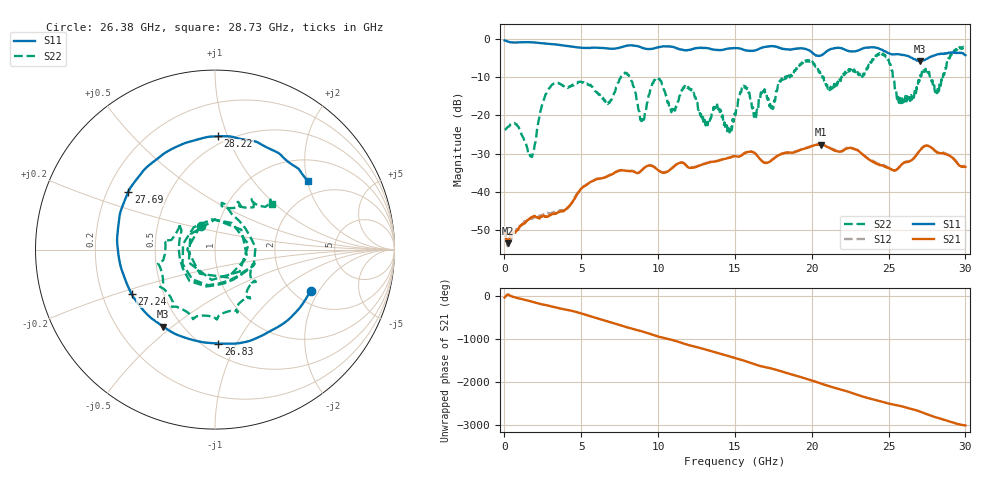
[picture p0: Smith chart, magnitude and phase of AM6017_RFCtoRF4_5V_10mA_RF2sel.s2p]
!Agilent Technologies,E8364B,MY43040894,A.07.50.67
!Agilent E8364B: A.07.50.67
!Date: Tuesday, August 21, 2018 13:31:20
!Correction: S11(Full 2 Port(1,2))
!S21(Full 2 Port(1,2))
!S12(Full 2 Port(1,2))
!S22(Full 2 Port(1,2))
!S2P File: Measurements: S11, S21, S12, S22:
# Hz S  dB  R 50
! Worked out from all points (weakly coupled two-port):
!   1601 points, 10 MHz to 30 GHz, reference 50 ohm
!   highest |S21| = -27.63 dB at 20.57 GHz (marker M1); lowest = -53.5 dB at 253.7 MHz (marker M2)
!   lowest |S11| = -5.7 dB at 27.06 GHz (marker M3), VSWR 3.14, Z = 19.9 - j23.2 ohm
!   |S11| at or under -10 dB: nowhere
!   |S22| runs from -30.9 to -1.7 dB; largest |S21 - S12| = 0.0061
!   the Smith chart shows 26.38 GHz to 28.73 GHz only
!   S11 on the Smith chart (normalised r, x): 26.38 GHz: 2.45, -1.69; 26.83 GHz: 0.59, -0.85; 27.24 GHz: 0.33, -0.22; 27.69 GHz: 0.29, +0.28; 28.22 GHz: 0.44, +0.92; 28.73 GHz: 1.55, +2.02
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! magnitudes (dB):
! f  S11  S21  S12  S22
! 10 MHz  -0.4  -50.1  -50.4  -23.7
! 253.7 MHz  -0.7  -53.5  -53.9  -23.0
! 1.772 GHz  -0.9  -46.7  -47.1  -30.9
! 2.934 GHz  -1.3  -46.2  -45.7  -12.8
! 5.015 GHz  -2.3  -39.1  -39.1  -11.2
! 6.739 GHz  -2.5  -35.9  -35.8  -17.0
! 7.957 GHz  -1.7  -34.6  -34.5  -8.9
! 8.97 GHz  -2.3  -34.2  -34.2  -21.9
! 10.02 GHz  -2.2  -34.4  -34.4  -10.4
! 10.96 GHz  -2.1  -33.6  -33.6  -19.0
! 15.01 GHz  -2.4  -30.7  -30.6  -19.9
! 20.01 GHz  -3.5  -28.1  -27.9  -6.1
! 20.57 GHz  -4.3  -27.6  -27.5  -9.3
! 25.01 GHz  -3.7  -33.9  -33.8  -5.5
! 26.38 GHz  -4.7  -32.0  -31.9  -16.1
! 26.83 GHz  -5.6  -30.3  -30.2  -12.6
! 27.06 GHz  -5.7  -29.1  -29.0  -9.5
! 27.24 GHz  -5.6  -28.4  -28.2  -9.0
! 27.69 GHz  -4.7  -28.2  -28.1  -9.8
! 28.22 GHz  -4.0  -29.8  -29.7  -12.9
! 28.73 GHz  -3.8  -30.1  -30.0  -7.8
! 30 GHz  -4.3  -33.5  -33.3  -1.7
